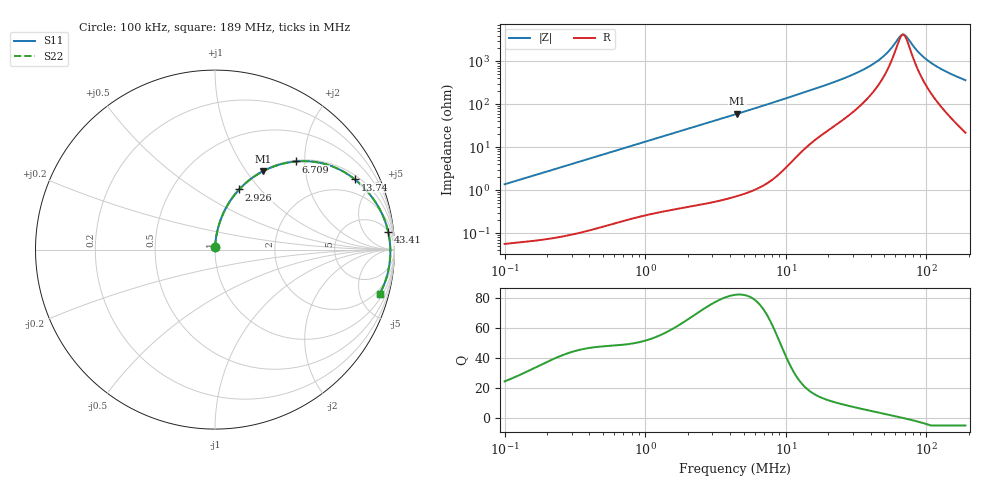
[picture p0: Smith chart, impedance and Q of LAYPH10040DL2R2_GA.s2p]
! LAYPH10040DL2R2_GA  S-PARAMETER MODEL  ( General Type )
! Model Generated by TAIYO YUDEN Corporation (http://www.ty-top.com)
! Version 1.0
! TAIYO YUDEN Control No. 180920NI43SB-FBB
! Copyright(c) 2018 TAIYO YUDEN CO.,LTD. All Rights Reserved.
! Product Description (link to TY-COMPAS)
! https://ds.yuden.co.jp/TYCOMPAS/or/detail?pn=LAYPH10040DL2R2NGA&u=M
! Products Name : Inductors
! Characteristics :
!  Inductance : 2.2 uH , SRF(min) : -Hz , DC Resistance(max) : 0.014 Ohm
!  Rated Current : Saturation :7.5 A , Temp Rise : 3.1 A (25 degC)
!  Case Size : 10.1 x 10.0 / 0.398 x 0.394 [mm/inch] , Thickness : 4 / 0.157 [mm/inch]
!  (Conditions: Temperature = 25 degC , DC Bias Current/Voltage = 0A / 0V)
! External Node Assignments :
!  1  o---GGG---o  2
! GND o---------o GND
! Frequency Range : 0.1MHz  -  189.042664MHz  [ 402 STEP ]
# MHz S RI R 50
! Freq[MHz].  S11 Real  S11 Imag  S21 Real  S21 Imag  S12 Real  S12 Imag  S22 Real  S22 Imag
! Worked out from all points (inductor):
!   401 points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, 100 kHz to 189 MHz, reference 50 ohm
!   read as one part in series: L = 2.18 uH near 103.8 kHz
!   highest Q = 82.3 at 4.515 MHz (marker M1), where L = 2.12 uH
!   self-resonance near 68.08 MHz
!   S11 on the Smith chart (normalised r, x): 100 kHz: 1.00, +0.03; 2.926 MHz: 1.01, +0.78; 6.709 MHz: 1.02, +1.81; 13.74 MHz: 1.19, +3.88; 43.41 MHz: 6, +18; 189 MHz: 1.44, -7.28
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0.1  0.000751 0.0137  0.9992 -0.0137  0.9992 -0.0137  0.000751 0.0137
0.353854  0.00334 0.0478  0.9967 -0.0478  0.9967 -0.0478  0.00334 0.0478
1.252125  0.0301 0.1619  0.9699 -0.1619  0.9699 -0.1619  0.0301 0.1619
2.925907  0.1349 0.3351  0.8651 -0.3351  0.8651 -0.3351  0.1349 0.3351
4.347904  0.2543 0.4294  0.7457 -0.4294  0.7457 -0.4294  0.2543 0.4294
4.515052  0.2689 0.4373  0.7311 -0.4373  0.7311 -0.4373  0.2689 0.4373
6.709376  0.4505 0.4909  0.5495 -0.4909  0.5495 -0.4909  0.4505 0.4909
9.245617  0.6143 0.4766  0.3857 -0.4766  0.3857 -0.4766  0.6143 0.4766
13.73901  0.7796 0.3908  0.2204 -0.3908  0.2204 -0.3908  0.7796 0.3908
15.38522  0.8143 0.3602  0.1857 -0.3602  0.1857 -0.3602  0.8143 0.3602
28.66948  0.9328 0.1946  0.0672 -0.1946  0.0672 -0.1946  0.9328 0.1946
35.95147  0.9539 0.1397  0.0461 -0.1397  0.0461 -0.1397  0.9539 0.1397
43.41409  0.9654 0.0967  0.0346 -0.0967  0.0346 -0.0967  0.9654 0.0967
54.44117  0.9737 0.0474  0.0263 -0.0474  0.0263 -0.0474  0.9737 0.0474
64.51342  0.9765 0.0114  0.0235 -0.0114  0.0235 -0.0114  0.9765 0.0114
66.99353  0.9768 0.00342  0.0232 -0.00342  0.0232 -0.00342  0.9768 0.00342
69.56898  0.977 -0.00457  0.023 0.00457  0.023 0.00457  0.977 -0.00457
73.61899  0.977 -0.0166  0.023 0.0166  0.023 0.0166  0.977 -0.0166
87.23936  0.9752 -0.0532  0.0248 0.0532  0.0248 0.0532  0.9752 -0.0532
103.3796  0.9705 -0.0912  0.0295 0.0912  0.0295 0.0912  0.9705 -0.0912
134.6216  0.9559 -0.1549  0.0441 0.1549  0.0441 0.1549  0.9559 -0.1549
189.0427  0.9173 -0.2469  0.0827 0.2469  0.0827 0.2469  0.9173 -0.2469
